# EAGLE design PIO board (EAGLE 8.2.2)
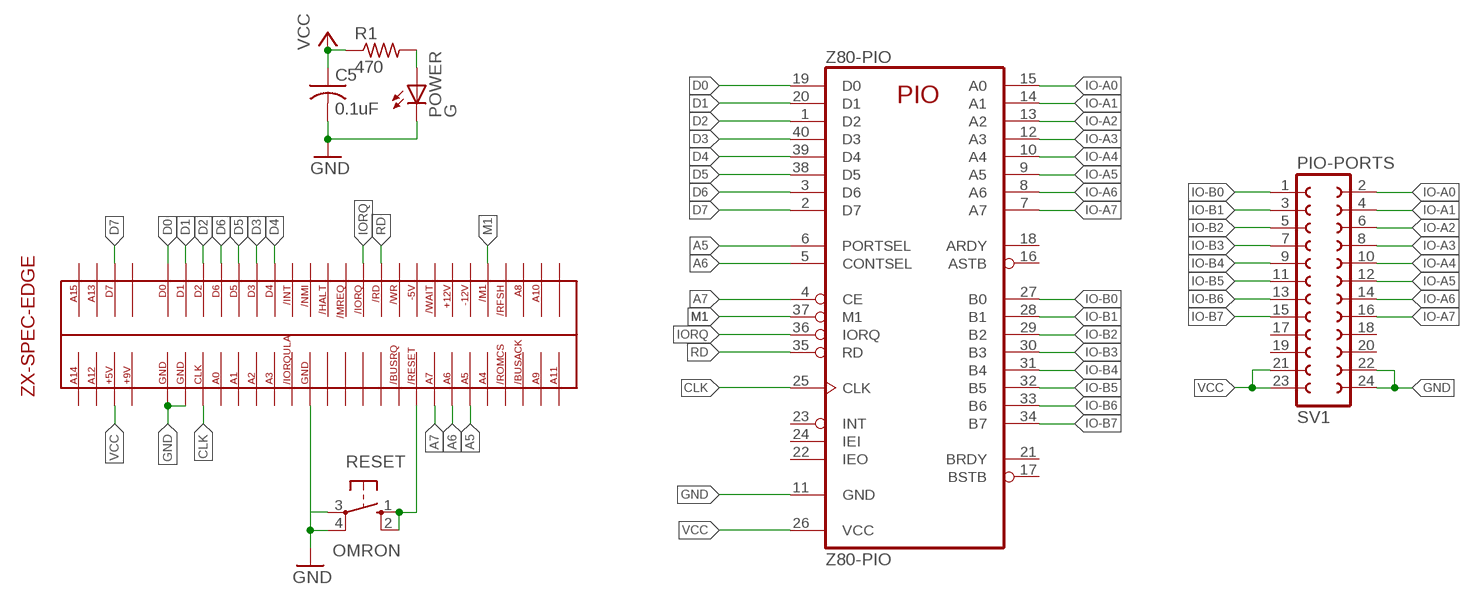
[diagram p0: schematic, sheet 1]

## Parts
1  ZX-EDGE-SPECCY  [ZX-EDGE-SPEC]
C5  0.1uF  C-US025-025X050  [C025-025X050]
POWER  G  LED5MM  [LED5MM]
R1  470  R-US_0207/7  [0207/7]
RESET  OMRON  10-XX  [B3F-10XX]
SV1  PIO-PORTS  FE12-2  [FE12-2]
Z80-PIO  Z80-PIO  Z80PIO  [DIL40]

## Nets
A5: 1.A5 Z80-PIO.6(PORTSEL)
A6: 1.A6 Z80-PIO.5(CONTSEL)
A7: 1.A7 Z80-PIO.4(CE)
CLK: 1.CLK Z80-PIO.25(CLK)
D0: 1.D0 Z80-PIO.19(D0)
D1: 1.D1 Z80-PIO.20(D1)
D2: 1.D2 Z80-PIO.1(D2)
D3: 1.D3 Z80-PIO.40(D3)
D4: 1.D4 Z80-PIO.39(D4)
D5: 1.D5 Z80-PIO.38(D5)
D6: 1.D6 Z80-PIO.3(D6)
D7: 1.D7 Z80-PIO.2(D7)
GND: 1.GND1 1.GND2 1.GND3 C5.2 POWER.K(C) RESET.3(P) RESET.4(P1) SV1.22 SV1.24 Z80-PIO.11(GND)
IO-A0: SV1.2 Z80-PIO.15(A0)
IO-A1: SV1.4 Z80-PIO.14(A1)
IO-A2: SV1.6 Z80-PIO.13(A2)
IO-A3: SV1.8 Z80-PIO.12(A3)
IO-A4: SV1.10 Z80-PIO.10(A4)
IO-A5: SV1.12 Z80-PIO.9(A5)
IO-A6: SV1.14 Z80-PIO.8(A6)
IO-A7: SV1.16 Z80-PIO.7(A7)
IO-B0: SV1.1 Z80-PIO.27(B0)
IO-B1: SV1.3 Z80-PIO.28(B1)
IO-B2: SV1.5 Z80-PIO.29(B2)
IO-B3: SV1.7 Z80-PIO.30(B3)
IO-B4: SV1.9 Z80-PIO.31(B4)
IO-B5: SV1.11 Z80-PIO.32(B5)
IO-B6: SV1.13 Z80-PIO.33(B6)
IO-B7: SV1.15 Z80-PIO.34(B7)
IORQ: 1./IORQ Z80-PIO.36(IORQ)
M1: 1./M1 Z80-PIO.37(M1)
N$1: 1./RST RESET.1(S) RESET.2(S1)
N$3: POWER.A R1.2
RD: 1./RD Z80-PIO.35(RD)
VCC: 1.+5 C5.1 R1.1 SV1.21 SV1.23 Z80-PIO.26(VCC)
Unconnected: 1.+9 1.+12 1.-5(-5V) 1.-12 1./BUSAK 1./BUSRQ 1./HALT 1./INT 1./IORQULA 1./MREQ 1./NMI 1./RFSH(/REFSH) 1./ROMCS 1./WAIT 1./WR 1.A0 1.A1 1.A2 1.A3 1.A4 1.A8 1.A9 1.A10 1.A11 1.A12 1.A13 1.A14 1.A15 1.N/C1 1.N/C2 1.N/C3 1.N/C4 1.N/C5 1.N/C6 SV1.17 SV1.18 SV1.19 SV1.20 Z80-PIO.16(ASTB) Z80-PIO.17(BSTB) Z80-PIO.18(ARDY) Z80-PIO.21(BRDY) Z80-PIO.22(IEO) Z80-PIO.23(INT) Z80-PIO.24(IEI)

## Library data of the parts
1 = sinclair-zx-spec:ZX-EDGE-SPECCY: ZX SPECTRUM EDGE CONNECTOR
C5 = rcl:C-US: CAPACITOR, American symbol
POWER = adafruit:LED: LED
R1 = adafruit:R-US_: RESISTOR, American symbol
RESET = switch-omron:10-XX: OMRON SWITCH; MPN: B3F-1000; OC_FARNELL: 176432; OC_NEWARK: 36M3542
SV1 = con-lsta:FE12-2: FEMALE HEADER; OC_FARNELL: unknown; OC_NEWARK: unknown
Z80-PIO = zilog:Z80PIO: Z80 FAMILY DEVICE

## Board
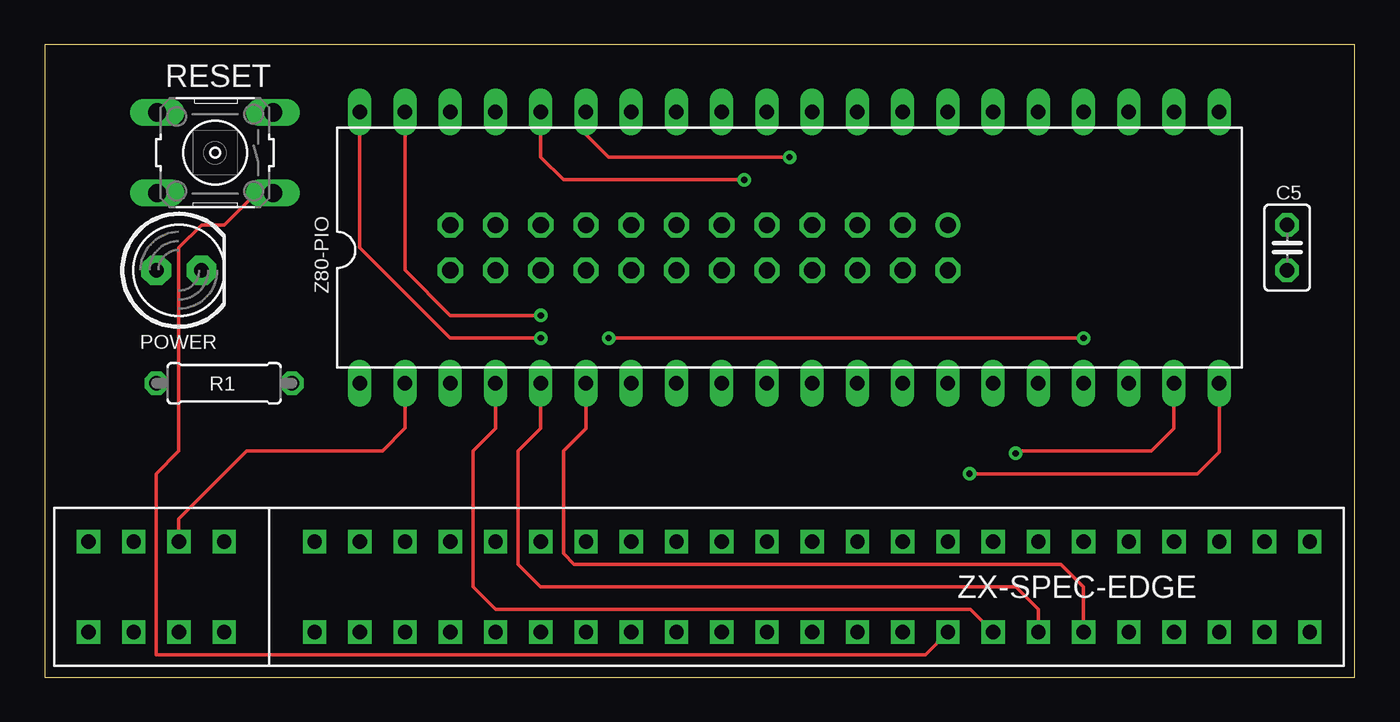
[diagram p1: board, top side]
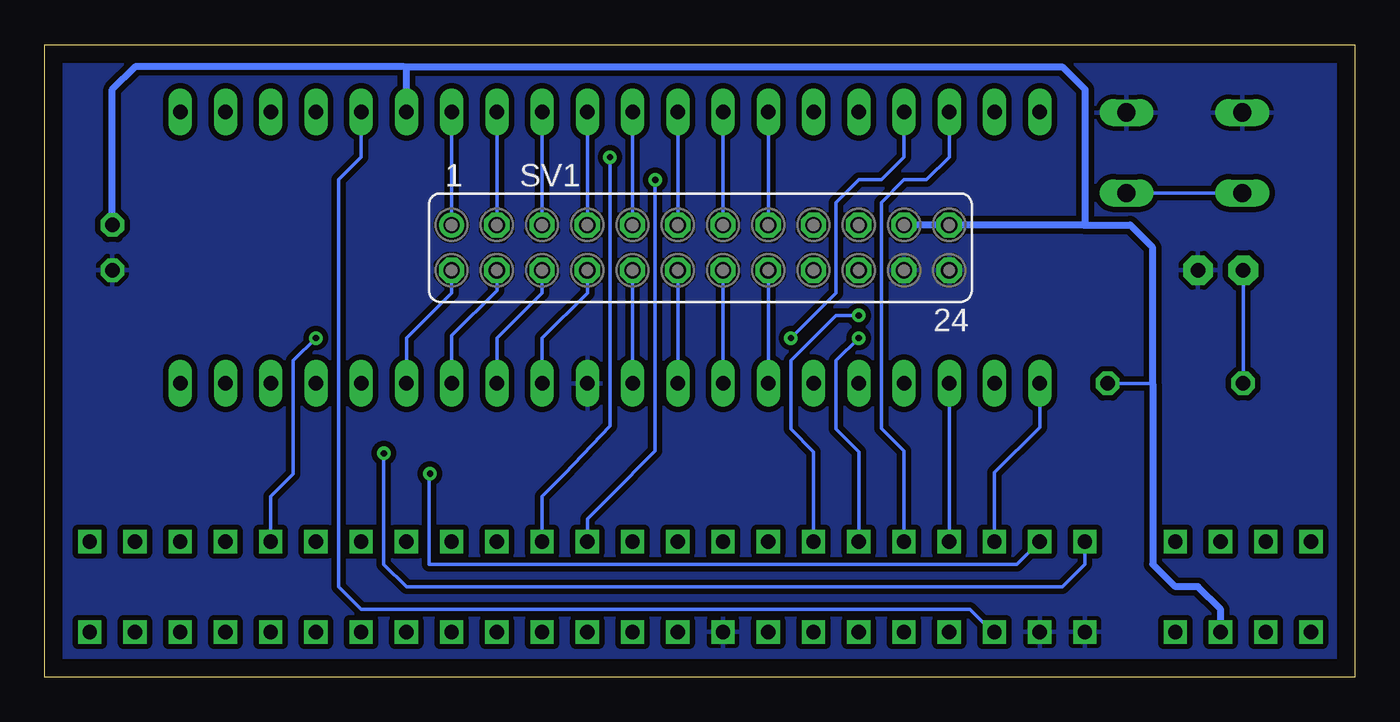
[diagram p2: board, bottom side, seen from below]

Size 73.58 x 35.54 mm. Coordinates in mm from the lower left corner, seen from the top.
Outline: 73.58,0 73.58,35.54 0,35.54 0,0 73.58,0
Copper layers (1*16): Top 0.035mm / dielectric 1.5mm / Bottom 0.035mm
Design rules "default *": minimum track width 6mil, minimum drill 0.35mm, track to track 6mil, track to pad 6mil, pad to pad 6mil, via to via 6mil, smd to smd 6mil, copper to edge 40mil, drill to drill 6mil, minimum pad ring 10mil, minimum via ring 8mil, stop-mask expansion 6mil, vias tented up to drill 0mil, thermal gap 10mil

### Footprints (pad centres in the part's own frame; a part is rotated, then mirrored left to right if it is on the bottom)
ZX-EDGE-SPEC = drill 0.8 square: +5 -5.08,-2.54; +9 -2.54,-2.54; +12 43.18,2.54; -5 38.1,2.54; -12 45.72,2.54; /BUSAK 53.34,-2.54; /BUSRQ 35.56,-2.54; /HALT 25.4,2.54; /INT 20.32,2.54; /IORQ 30.48,2.54; /IORQULA 20.32,-2.54; /M1 48.26,2.54; /MREQ 27.94,2.54; /NMI 22.86,2.54; /RD 33.02,2.54; /RFSH 50.8,2.54; /ROMCS 50.8,-2.54; /RST 38.1,-2.54; /WAIT 40.64,2.54; /WR 35.56,2.54; A0 10.16,-2.54; A1 12.7,-2.54; A2 15.24,-2.54; A3 17.78,-2.54; A4 48.26,-2.54; A5 45.72,-2.54; A6 43.18,-2.54; A7 40.64,-2.54; A8 53.34,2.54; A9 55.88,-2.54; A10 55.88,2.54; A11 58.42,-2.54; A12 -7.62,-2.54; A13 -7.62,2.54; A14 -10.16,-2.54; A15 -10.16,2.54; CLK 7.62,-2.54; D0 2.54,2.54; D1 5.08,2.54; D2 7.62,2.54; D3 15.24,2.54; D4 17.78,2.54; D5 12.7,2.54; D6 10.16,2.54; D7 -5.08,2.54; GND1 2.54,-2.54; GND2 5.08,-2.54; GND3 22.86,-2.54; N/C1 -2.54,2.54; N/C2 58.42,2.54; N/C3 25.4,-2.54; N/C4 27.94,-2.54; N/C5 30.48,-2.54; N/C6 33.02,-2.54
C025-025X050 = drill 0.813 octagon: 1 -1.27,0; 2 1.27,0
LED5MM = drill 0.813 pad 1.676 octagon: A -1.27,0; K 1.27,0
0207/7 = drill 0.813 octagon: 1 -3.81,0; 2 3.81,0
B3F-10XX = drill 1.016 long: 1 -3.251,2.261; 2 3.251,2.261; 3 -3.251,-2.261; 4 3.251,-2.261
FE12-2 = drill 0.914: 1 -13.97,1.27 | drill 0.914 octagon: 2 -13.97,-1.27; 3 -11.43,1.27; 4 -11.43,-1.27; 5 -8.89,1.27; 6 -8.89,-1.27; 7 -6.35,1.27; 8 -6.35,-1.27; 9 -3.81,1.27; 10 -3.81,-1.27; 11 -1.27,1.27; 12 -1.27,-1.27; 13 1.27,1.27; 14 1.27,-1.27; 15 3.81,1.27; 16 3.81,-1.27; 17 6.35,1.27; 18 6.35,-1.27; 19 8.89,1.27; 20 8.89,-1.27; 21 11.43,1.27; 22 11.43,-1.27; 23 13.97,1.27; 24 13.97,-1.27
DIL40 = drill 0.813 long: 1 -24.13,-7.62; 2 -21.59,-7.62; 3 -19.05,-7.62; 4 -16.51,-7.62; 5 -13.97,-7.62; 6 -11.43,-7.62; 7 -8.89,-7.62; 8 -6.35,-7.62; 9 -3.81,-7.62; 10 -1.27,-7.62; 11 1.27,-7.62; 12 3.81,-7.62; 13 6.35,-7.62; 14 8.89,-7.62; 15 11.43,-7.62; 16 13.97,-7.62; 17 16.51,-7.62; 18 19.05,-7.62; 19 21.59,-7.62; 20 24.13,-7.62; 21 24.13,7.62; 22 21.59,7.62; 23 19.05,7.62; 24 16.51,7.62; 25 13.97,7.62; 26 11.43,7.62; 27 8.89,7.62; 28 6.35,7.62; 29 3.81,7.62; 30 1.27,7.62; 31 -1.27,7.62; 32 -3.81,7.62; 33 -6.35,7.62; 34 -8.89,7.62; 35 -11.43,7.62; 36 -13.97,7.62; 37 -16.51,7.62; 38 -19.05,7.62; 39 -21.59,7.62; 40 -24.13,7.62

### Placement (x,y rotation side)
1  12.62,5.08 0 top
C5  69.77,24.13 270 top
POWER  7.54,22.86 0 top
R1  10.08,16.51 180 top
RESET  9.58,29.46 180 top
SV1  36.75,24.13 0 bottom
Z80-PIO  41.83,24.13 0 top

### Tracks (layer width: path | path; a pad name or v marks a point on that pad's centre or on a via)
A5
  Top 0.2: Z80-PIO.6 30.4,13.97 29.13,12.7 29.13,6.96 29.74,6.35 57.07,6.35 58.34,5.08 1.A5
A6
  Top 0.2: Z80-PIO.5 27.86,13.97 26.59,12.7 26.59,6.35 27.86,5.08 54.53,5.08 55.8,3.81 1.A6
A7
  Top 0.2: 51.99,3.81 25.32,3.81 24.05,5.08 24.05,12.7 25.32,13.97 Z80-PIO.4
  Top 0.203: 1.A7 51.99,3.81
CLK
  Bottom 0.2: Z80-PIO.25 55.8,29.21 57.07,27.94 57.07,5.08 55.8,3.81 21.62,3.81
  Bottom 0.203: 1.CLK 20.35,2.54 21.62,3.81
D0  (via drill 0.35)
  Top 0.2: Z80-PIO.19 63.42,13.97 62.15,12.7 54.53,12.7 v54.53,12.58
  Bottom 0.2: v54.53,12.58 54.53,6.35 53.26,5.08 16.43,5.08 15.16,6.35 1.D0
D1  (via drill 0.35)
  Top 0.2: v51.94,11.43 64.74,11.43 65.96,12.65 Z80-PIO.20
  Bottom 0.2: 1.D1 18.97,6.35 29.13,6.35
  Bottom 0.203: 29.13,6.35 51.99,6.35 51.99,11.43 v51.94,11.43
D2
  Bottom 0.203: Z80-PIO.1 17.7,14.03 20.24,11.49 1.D2
D3  (via drill 0.35)
  Top 0.203: v27.86,19.05 22.78,19.05 17.7,24.13 Z80-PIO.40
  Bottom 0.2: 1.D3 27.86,12.67 29.13,13.94 29.13,17.78
  Bottom 0.203: 29.13,17.78 v27.86,19.05
D4  (via drill 0.35)
  Top 0.203: v27.86,20.32 22.78,20.32 20.24,22.86 Z80-PIO.39
  Bottom 0.2: 1.D4 30.4,12.67 31.67,13.94 31.67,17.78
  Bottom 0.203: 31.67,17.78 29.13,20.32 v27.86,20.32
D5
  Bottom 0.203: 1.D5 25.32,12.7 26.59,13.97 26.59,26.67 25.32,27.94 24.05,27.94 22.78,29.21 Z80-PIO.38
D6
  Bottom 0.2: 1.D6 Z80-PIO.3
D7
  Top 0.203: Z80-PIO.2 20.24,13.99 18.97,12.72 18.97,12.7 11.35,12.7 7.54,8.89 1.D7
GND
  pour Bottom (isolate 0.305): -0.08,0 -0.08,35.56 73.58,35.56 73.58,0
IO-A0
  Bottom 0.2: Z80-PIO.15 53.26,19.06 50.74,21.59 50.72,21.59 SV1.2
IO-A1
  Bottom 0.2: SV1.4 48.18,21.72 50.72,19.18 Z80-PIO.14
IO-A2
  Bottom 0.2: SV1.6 45.64,21.59 48.18,19.05 Z80-PIO.13
IO-A3
  Bottom 0.2: Z80-PIO.12 45.64,19.05 43.1,21.59 SV1.8
IO-A4
  Bottom 0.2: Z80-PIO.10 SV1.10
IO-A5
  Bottom 0.2: Z80-PIO.9 SV1.12
IO-A6
  Bottom 0.2: Z80-PIO.8 SV1.14
IO-A7
  Bottom 0.2: Z80-PIO.7 SV1.16
IO-B0
  Bottom 0.2: SV1.1 Z80-PIO.27
IO-B1
  Bottom 0.2: SV1.3 Z80-PIO.28
IO-B2
  Bottom 0.2: SV1.5 Z80-PIO.29
IO-B3
  Bottom 0.2: SV1.7 Z80-PIO.30
IO-B4
  Bottom 0.2: SV1.9 Z80-PIO.31
IO-B5
  Bottom 0.2: SV1.11 Z80-PIO.32
IO-B6
  Bottom 0.2: SV1.13 Z80-PIO.33
IO-B7
  Bottom 0.2: SV1.15 Z80-PIO.34
IORQ  (via drill 0.35)
  Top 0.2: v39.29,27.94 29.13,27.94 27.86,29.21 Z80-PIO.36
  Bottom 0.2: 39.29,12.7 v39.29,27.94 | 41.83,10.16 43.1,8.89 1./IORQ
  Bottom 0.203: 41.83,10.16 39.29,12.7
M1  (via drill 0.35)
  Top 0.203: v58.34,19.05 v31.67,19.05
  Bottom 0.203: 1./M1 60.88,10.16 59.61,11.43 59.61,17.78 v58.34,19.05 | v31.67,19.05 29.13,21.59 29.13,26.67 27.86,27.94 26.59,27.94 25.32,29.21 Z80-PIO.37
N$1
  Top 0.203: RESET.1 11.89,27.2 10.08,25.4 8.81,25.4 7.54,24.13 7.54,12.7 6.27,11.43 6.27,1.27 49.45,1.27 1./RST
  Bottom 0.203: RESET.2 RESET.1
N$3
  Bottom 0.203: POWER.A R1.2
RD  (via drill 0.35)
  Top 0.203: v41.83,29.21 31.67,29.21 30.4,30.48 Z80-PIO.35
  Bottom 0.203: v41.83,29.21 41.83,14.1 44.37,11.43 45.64,10.16 1./RD
VCC
  Bottom 0.203: R1.1 11.38,16.51 11.35,16.48
  Bottom 0.406: SV1.21 SV1.23 15.26,25.4 | 1.+5 7.54,3.81 8.81,5.08 10.08,5.08 11.35,6.35 11.35,16.48 11.35,24.13 12.62,25.4 15.26,25.4 | C5.1 69.77,33.02 68.5,34.29 53.39,34.29 | 53.39,34.29 16.43,34.29 15.16,33.02 15.16,25.5 15.26,25.4 | Z80-PIO.26 53.26,34.16 53.39,34.29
